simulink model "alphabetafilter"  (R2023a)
settings: Solver=ode1  StartTime=0.0  StopTime=10.0  FixedStep=Ts  RelTol=1e-3
PreLoadFcn:
  | Ts = 0.001;
  | dt = 0.01;
  | Q = 1e-3;
  | R = 1e-4;

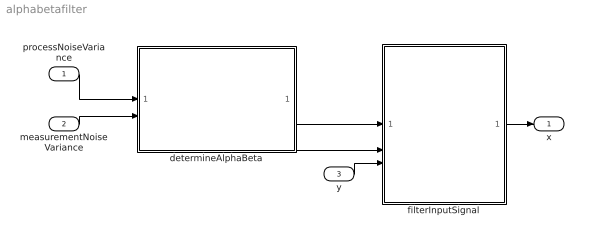
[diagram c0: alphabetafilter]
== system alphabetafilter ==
  processNoiseVariance : Inport
  measurementNoiseVariance : Inport  Port=2
  y : Inport  Port=3
  determineAlphaBeta : Subsystem
  filterInputSignal : Subsystem
  x : Outport
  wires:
  measurementNoiseVariance/1 -> determineAlphaBeta/2(measurementNoiseVariance)
  processNoiseVariance/1 -> determineAlphaBeta/1(processNoiseVariance)
  determineAlphaBeta/1(alpha) -> filterInputSignal/1(alpha)
  determineAlphaBeta/2(beta) -> filterInputSignal/2(beta)
  y/1 -> filterInputSignal/3(y)
  filterInputSignal/1(x) -> x/1

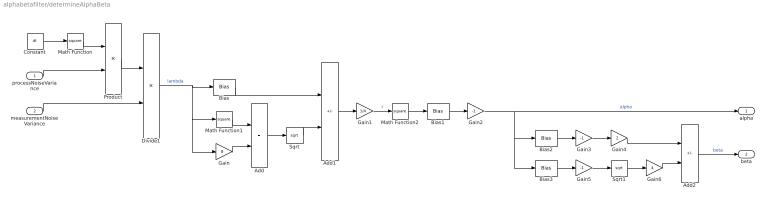
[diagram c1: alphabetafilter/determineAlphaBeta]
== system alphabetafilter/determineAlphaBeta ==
  processNoiseVariance : Inport
  measurementNoiseVariance : Inport  Port=2
  Add : Sum
  Add1 : Sum  Inputs=+-
  Add2 : Sum  Inputs=+-
  Bias : Bias  Bias=4
  Bias1 : Bias  Bias=-1
  Bias2 : Bias  Bias=-2
  Bias3 : Bias  Bias=-1
  Constant : Constant  Value=dt
  Divide1 : Product  Inputs=*/
  Gain : Gain  Gain=8
  Gain1 : Gain  Gain=1/4
  Gain2 : Gain  Gain=-1
  Gain3 : Gain  Gain=-1
  Gain4 : Gain  Gain=2
  Gain5 : Gain  Gain=-1
  Gain6 : Gain  Gain=4
  Math Function : Math  Operator=square
  Math Function1 : Math  Operator=square
  Math Function2 : Math  Operator=square
  Product : Product
  Sqrt : Sqrt
  Sqrt1 : Sqrt
  alpha : Outport
  beta : Outport  Port=2
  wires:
  Add/1 -> Sqrt/1
  Math Function2/1 -> Bias1/1
  Gain1/1 -> Math Function2/1  "r"
  Sqrt/1 -> Add1/2
  Bias/1 -> Add1/1
  Bias1/1 -> Gain2/1
  Add2/1 -> beta/1  "beta"
  Math Function/1 -> Product/1
  Gain5/1 -> Sqrt1/1
  Add1/1 -> Gain1/1
  Bias3/1 -> Gain5/1
  Divide1/1 -> Bias/1, Gain/1, Math Function1/1  "lambda"
  Bias2/1 -> Gain3/1
  Product/1 -> Divide1/1
  Gain/1 -> Add/2
  Sqrt1/1 -> Gain6/1
  Gain2/1 -> Bias3/1, Bias2/1, alpha/1  "alpha"
  Gain3/1 -> Gain4/1
  Gain6/1 -> Add2/2
  Math Function1/1 -> Add/1
  Gain4/1 -> Add2/1
  Constant/1 -> Math Function/1
  measurementNoiseVariance/1 -> Divide1/2
  processNoiseVariance/1 -> Product/2

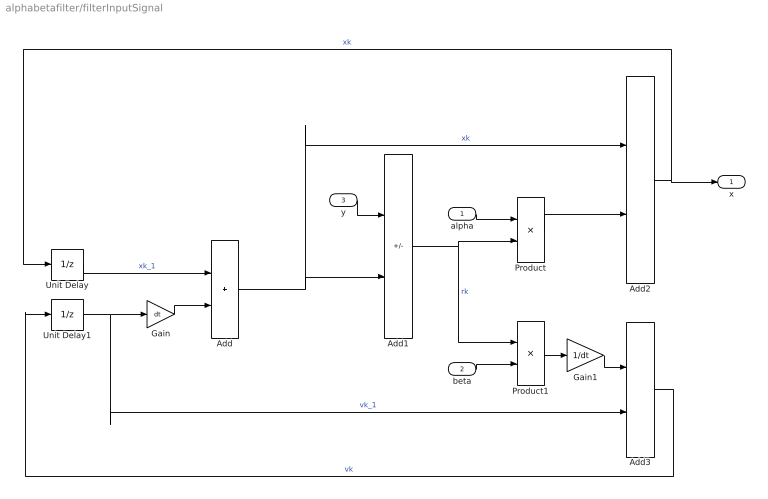
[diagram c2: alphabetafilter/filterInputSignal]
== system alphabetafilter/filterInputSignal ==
  alpha : Inport
  beta : Inport  Port=2
  y : Inport  Port=3
  Add : Sum
  Add1 : Sum  Inputs=+-
  Add2 : Sum
  Add3 : Sum
  Gain : Gain  Gain=dt
  Gain1 : Gain  Gain=1/dt
  Product : Product
  Product1 : Product
  Unit Delay : UnitDelay  SampleTime=-1  HasFrameUpgradeWarning=on
  Unit Delay1 : UnitDelay  SampleTime=-1  HasFrameUpgradeWarning=on
  x : Outport
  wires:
  Add1/1 -> Product1/1, Product/2  "rk"
  Unit Delay/1 -> Add/1  "xk_1"
  Add3/1 -> Unit Delay1/1  "vk"
  Unit Delay1/1 -> Gain/1, Add3/2  "vk_1"
  y/1 -> Add1/1
  Product/1 -> Add2/2
  Add2/1 -> x/1, Unit Delay/1  "xk"
  Gain1/1 -> Add3/1
  Product1/1 -> Gain1/1
  alpha/1 -> Product/1
  Gain/1 -> Add/2
  Add/1 -> Add1/2, Add2/1  "xk"
  beta/1 -> Product1/2
